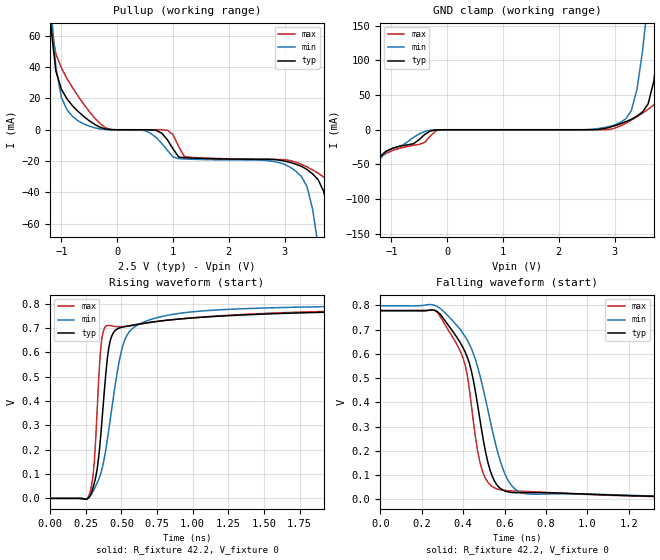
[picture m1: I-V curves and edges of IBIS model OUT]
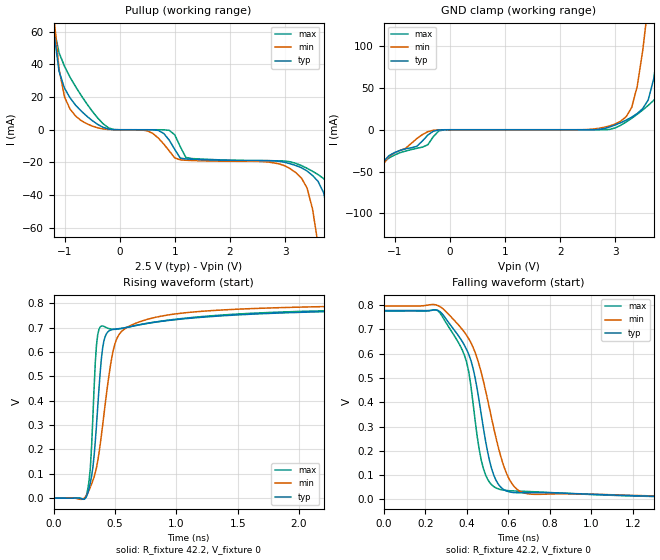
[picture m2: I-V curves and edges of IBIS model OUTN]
|   IBIS File of SG2520HHN D
|   HCSL Zdiff=85, Vcc=2.5V, fo<=212.5MHz
[IBIS Ver]   3.2
[File Name]   sg2520hhn_85_25v.ibs
[File Rev]   1.0
[Date]   Jan. 27, 2023
[Source]
[Notes]
Created by Minoru Kozaki
[Disclaimer]
Seiko Epson Corporation makes no warranty with respect to the
information contained herein.
[Copyright]
Copyright(C) 2023, Seiko Epson Corporation. All rights reserved.
|   Component
[Component]   SG2520HHN
[Manufacturer]  Seiko Epson Corporation
[Package]
R_pkg   17.7m   NA   NA
L_pkg   235p   NA   NA
C_pkg   208f   NA   NA
[Pin]   signal_name   model_name   R_pin   L_pin   C_pin
1   OE/ST   NC
2   NC   NC
3   GND   GND
4   OUT   OUT   17.7m   235p   208f
5   OUTN   OUTN   10.4m   129p   221f
6   VCC   POWER
[Diff Pin] inv_pin  vdiff  tdelay_typ
4   5   0   0
| Models and submodels in the file (2): OUT (Open_source), OUTN (Open_source)
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|   Model OUT
[Model]   OUT
Model_type   Open_source
Polarity   Non-Inverting
Vref = 0
Vmeas = 0.4
Rref = 42.2
Cref = 0
C_comp   12.0p   12.0p   12.0p
[Temperature Range]   25   105   -40
[Voltage Range]   2.5   2.25   2.75
[Pullup Reference]   2.5   2.25   2.75
[GND Clamp Reference]   0   0   0
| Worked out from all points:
|   GND clamp passes 1 mA (typ) near -0.25 V on its own axis
|   falling waveform, R_fixture 42.2, V_fixture 0: 20-80 % time 117ps typ, 148ps min, 101ps max; typ from 0.777 V to 0 V
|   rising waveform, R_fixture 42.2, V_fixture 0: 20-80 % time 74.9ps typ, 138ps min, 46ps max; typ from 0 V to 0.776 V
[Pullup]
-2.5V     1.183A     1.136A     1.251A
-1.2V     69.64mA    83.39mA    69.73mA
-1V       25.77mA    20.56mA    39.44mA
-600mV    8.482mA    3.742mA    16.3mA
-200mV    363.3uA    114uA      1.084mA
900mV     -6.47mA    -13.13mA   -383.4uA
1.2V      -17.85mA   -18.64mA   -17.01mA
3.2V      -22.01mA   -26.45mA   -20.67mA
3.6V      -31.93mA   -74.43mA   -27.72mA
3.9V      -84.68mA   -152.4mA   -38.04mA
4.1V      -141.5mA   -204.4mA   -69.72mA
5V        -397.3mA   -439.1mA   -346.2mA
[GND Clamp]
-2.5V     -395.8mA   -372.8mA   -422.3mA
-1.7V     -168.7mA   -164.6mA   -175.3mA
-1.6V     -140.3mA   -138.7mA   -144.5mA
-1.2V     -38.58mA   -41.69mA   -39.96mA
-400mV    -6.528mA   -2.401mA   -18.23mA
3.1V      8.482mA    10.36mA    5.398mA
3.3V      15.19mA    28.06mA    13.89mA
3.6V      37.47mA    189.3mA    29.64mA
3.8V      132.2mA    347.8mA    43.46mA
3.9V      214.1mA    427.7mA    56.09mA
4.1V      385.8mA    588.6mA    162.9mA
5V        1.183A     1.404A     1.01A
[Falling Waveform]
R_fixture = 42.2
V_fixture = 0
V_fixture_min = 0
V_fixture_max = 0
0s        776.9mV    797.6mV    778.9mV
260ps     779.9mV    800.4mV    779.8mV
390ps     639.8mV    695mV      603.2mV
440ps     528.2mV    620.9mV    385.8mV
470ps     388.3mV    545.7mV    199.1mV
500ps     231.9mV    443mV      100.8mV
540ps     96.21mV    288mV      53.06mV
600ps     35.17mV    108.3mV    37.21mV
690ps     27.69mV    25.83mV    33.19mV
4ns       332uV      516uV      248uV
[Rising Waveform]
R_fixture = 42.2
V_fixture = 0
V_fixture_min = 0
V_fixture_max = 0
0s        120uV      185uV      100uV
280ps     11mV       10.36mV    26.66mV
310ps     64.64mV    40.3mV     156.9mV
340ps     170.3mV    78.44mV    491.3mV
360ps     298.2mV    113.8mV    648.3mV
400ps     571.8mV    238.4mV    710.3mV
440ps     677.6mV    403.2mV    707.8mV
520ps     705.2mV    646.4mV    706.4mV
750ps     727.2mV    742.7mV    726.8mV
4ns       776mV      796.5mV    778.3mV
[Ramp]
R_load = 42.2
dV/dt_r   0.47324/76.95p   0.48533/142.26p   0.47511/46.85p
dV/dt_f   0.47324/122.32p   0.48533/152.26p   0.47511/106.63p
|   Model OUTN
[Model]   OUTN
Model_type   Open_source
Polarity   Inverting
Vref = 0
Vmeas = 0.4
Rref = 42.2
Cref = 0
C_comp   12.0p   12.0p   12.0p
[Temperature Range]   25   105   -40
[Voltage Range]   2.5   2.25   2.75
[Pullup Reference]   2.5   2.25   2.75
[GND Clamp Reference]   0   0   0
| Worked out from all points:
|   GND clamp passes 1 mA (typ) near -0.25 V on its own axis
|   falling waveform, R_fixture 42.2, V_fixture 0: 20-80 % time 114ps typ, 145ps min, 97.2ps max; typ from 0.776 V to 0 V
|   rising waveform, R_fixture 42.2, V_fixture 0: 20-80 % time 74.7ps typ, 140ps min, 45.6ps max; typ from 0 V to 0.774 V
[Pullup]
-2.5V     905.1mA    874.7mA    940.7mA
-1.2V     61.06mA    71.38mA    63.41mA
-1V       25.32mA    20mA       38.73mA
-600mV    8.406mA    3.724mA    16.07mA
-200mV    362.6uA    113.9uA    1.078mA
900mV     -6.359mA   -12.94mA   -382.1uA
1.2V      -17.84mA   -18.63mA   -16.92mA
3.2V      -21.9mA    -26.31mA   -20.58mA
3.6V      -31.53mA   -70.06mA   -27.38mA
3.9V      -79.2mA    -143.6mA   -37.3mA
4.1V      -132.5mA   -192.7mA   -65.08mA
5V        -372.4mA   -414mA     -322.6mA
[GND Clamp]
-2.5V     -371mA     -351.5mA   -393.4mA
-1.6V     -131.4mA   -130.7mA   -134.5mA
-1.2V     -37.5mA    -40.37mA   -38.88mA
-400mV    -6.389mA   -2.379mA   -17.99mA
-100mV    -21.28uA   -12.91uA   -96.74uA
3.1V      8.406mA    10.28mA    5.341mA
3.3V      15.03mA    26.75mA    13.7mA
3.6V      35.7mA     150.5mA    29.15mA
3.8V      107.2mA    274.3mA    42.57mA
3.9V      167.1mA    336.7mA    53.3mA
4.1V      298.5mA    462.2mA    129.2mA
5V        905.1mA    1.039A     760.1mA
[Falling Waveform]
R_fixture = 42.2
V_fixture = 0
V_fixture_min = 0
V_fixture_max = 0
0s        775.6mV    796.1mV    777.4mV
260ps     778.5mV    798.3mV    777mV
390ps     632.3mV    686.6mV    589.9mV
430ps     540.3mV    626.4mV    396.6mV
460ps     402mV      552.4mV    203.9mV
490ps     242.1mV    449.5mV    101.6mV
530ps     99.56mV    292.5mV    52.55mV
590ps     34.97mV    109.6mV    36.77mV
680ps     27.35mV    25.38mV    33.03mV
4ns       326uV      505uV      244uV
[Rising Waveform]
R_fixture = 42.2
V_fixture = 0
V_fixture_min = 0
V_fixture_max = 0
0s        111uV      187uV      99uV
270ps     8.467mV    12.43mV    15.11mV
300ps     64.14mV    45.72mV    125.4mV
330ps     170.9mV    86.32mV    446.7mV
350ps     299.9mV    125.5mV    628.1mV
390ps     573.1mV    258mV      706.4mV
430ps     673.7mV    422.6mV    700.1mV
510ps     694.4mV    647.6mV    693mV
750ps     715.9mV    731.6mV    716.6mV
4ns       774.5mV    794.7mV    776.7mV
[Ramp]
R_load = 42.2
dV/dt_r   0.47310/77.36p   0.48519/146.24p   0.47494/46.60p
dV/dt_f   0.47310/118.96p   0.48519/150.10p   0.47494/102.82p
